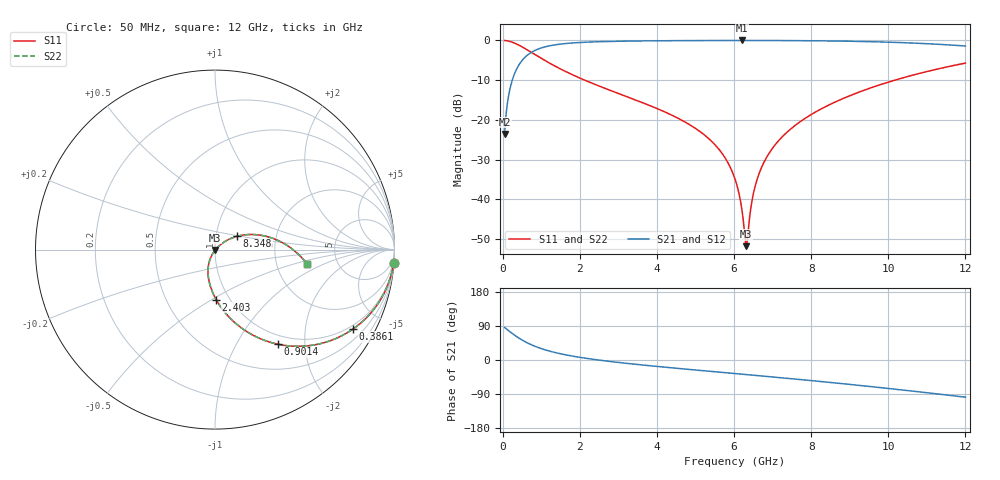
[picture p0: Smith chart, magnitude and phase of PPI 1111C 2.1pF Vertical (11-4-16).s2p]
# GHz S MA R 50
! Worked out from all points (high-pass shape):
!   1601 points, 50 MHz to 12 GHz, reference 50 ohm
!   highest |S21| = -0.03 dB at 6.212 GHz (marker M1); lowest = -23.5 dB at 50 MHz (marker M2)
!   |S21| within 3 dB of the highest: 741.4 MHz to end of sweep
!   lowest |S11| = -51.7 dB at 6.316 GHz (marker M3), VSWR 1.01, Z = 50.2 - j0.169 ohm
!   |S11| at or under -10 dB: 2.128 GHz to 10.17 GHz (8.044 GHz wide, 131 % of centre)
!   |S22| runs from -51.7 to 0.0 dB; largest |S21 - S12| = 0
!   S11 on the Smith chart (normalised r, x): 50 MHz: 1, -28; 386.1 MHz: 0.85, -3.57; 901.4 MHz: 0.86, -1.51; 2.403 GHz: 0.87, -0.52; 8.348 GHz: 1.27, +0.19; 12 GHz: 2.99, -0.64
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0.05  0.9978 -4.1  0.0668 85.8  0.0668 85.8  0.9978 -4.1
0.1919063  0.9685 -15.6  0.2489 74.4  0.2489 74.4  0.9685 -15.6
0.3860938  0.8879 -29.8  0.4596 60.2  0.4596 60.2  0.8879 -29.8
0.9014375  0.6347 -56.2  0.7719 33.7  0.7719 33.7  0.6347 -56.2
1.386906  0.4667 -70.8  0.8832 19.0  0.8832 19.0  0.4667 -70.8
2.044156  0.3291 -83.5  0.9428 6.3  0.9428 6.3  0.3291 -83.5
2.402656  0.2786 -88.7  0.9588 1.0  0.9588 1.0  0.2786 -88.7
4.038312  0.1367 -106.5  0.9885 -17.3  0.9885 -17.3  0.1367 -106.5
5.360281  0.05725 -117.4  0.9958 -29.7  0.9958 -29.7  0.05725 -117.4
5.756125  0.03407 -119.3  0.9967 -33.3  0.9967 -33.3  0.03407 -119.3
6.025  0.01809 -117.9  0.997 -35.8  0.997 -35.8  0.01809 -117.9
6.211719  0.007026 -106.2  0.9971 -37.5  0.9971 -37.5  0.007026 -106.2
6.278937  0.003522 -81.2  0.9971 -38.1  0.9971 -38.1  0.003522 -81.2
6.316281  0.002588 -40.5  0.9971 -38.4  0.9971 -38.4  0.002588 -40.5
6.353625  0.003426 1.8  0.997 -38.8  0.997 -38.8  0.003426 1.8
6.540344  0.01424 38.7  0.9969 -40.5  0.9969 -40.5  0.01424 38.7
6.809219  0.0315 42.0  0.9964 -43.0  0.9964 -43.0  0.0315 42.0
7.294688  0.06448 39.8  0.9946 -47.5  0.9946 -47.5  0.06448 39.8
8.019156  0.1183 33.9  0.9893 -54.5  0.9893 -54.5  0.1183 33.9
8.347781  0.1448 30.9  0.9856 -57.7  0.9856 -57.7  0.1448 30.9
10.01331  0.2998 14.0  0.9493 -75.2  0.9493 -75.2  0.2998 14.0
12  0.5177 -8.7  0.8497 -98.1  0.8497 -98.1  0.5177 -8.7
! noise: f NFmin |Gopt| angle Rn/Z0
0.05  0.0006779  0.9431  2.293  0.002667
1.372  0.004083  0.6993  10.7  0.002635
2.701  0.006433  0.6404  18.48  0.003296
4.031  0.008551  0.6117  26.12  0.00389
5.36  0.01061  0.5995  33.43  0.0045
6.682  0.0127  0.5986  40.3  0.005173
8.012  0.01492  0.6064  46.79  0.00597
9.341  0.01733  0.6213  52.87  0.006943
10.67  0.02004  0.6421  58.57  0.008172
12  0.02314  0.6675  63.97  0.009763
